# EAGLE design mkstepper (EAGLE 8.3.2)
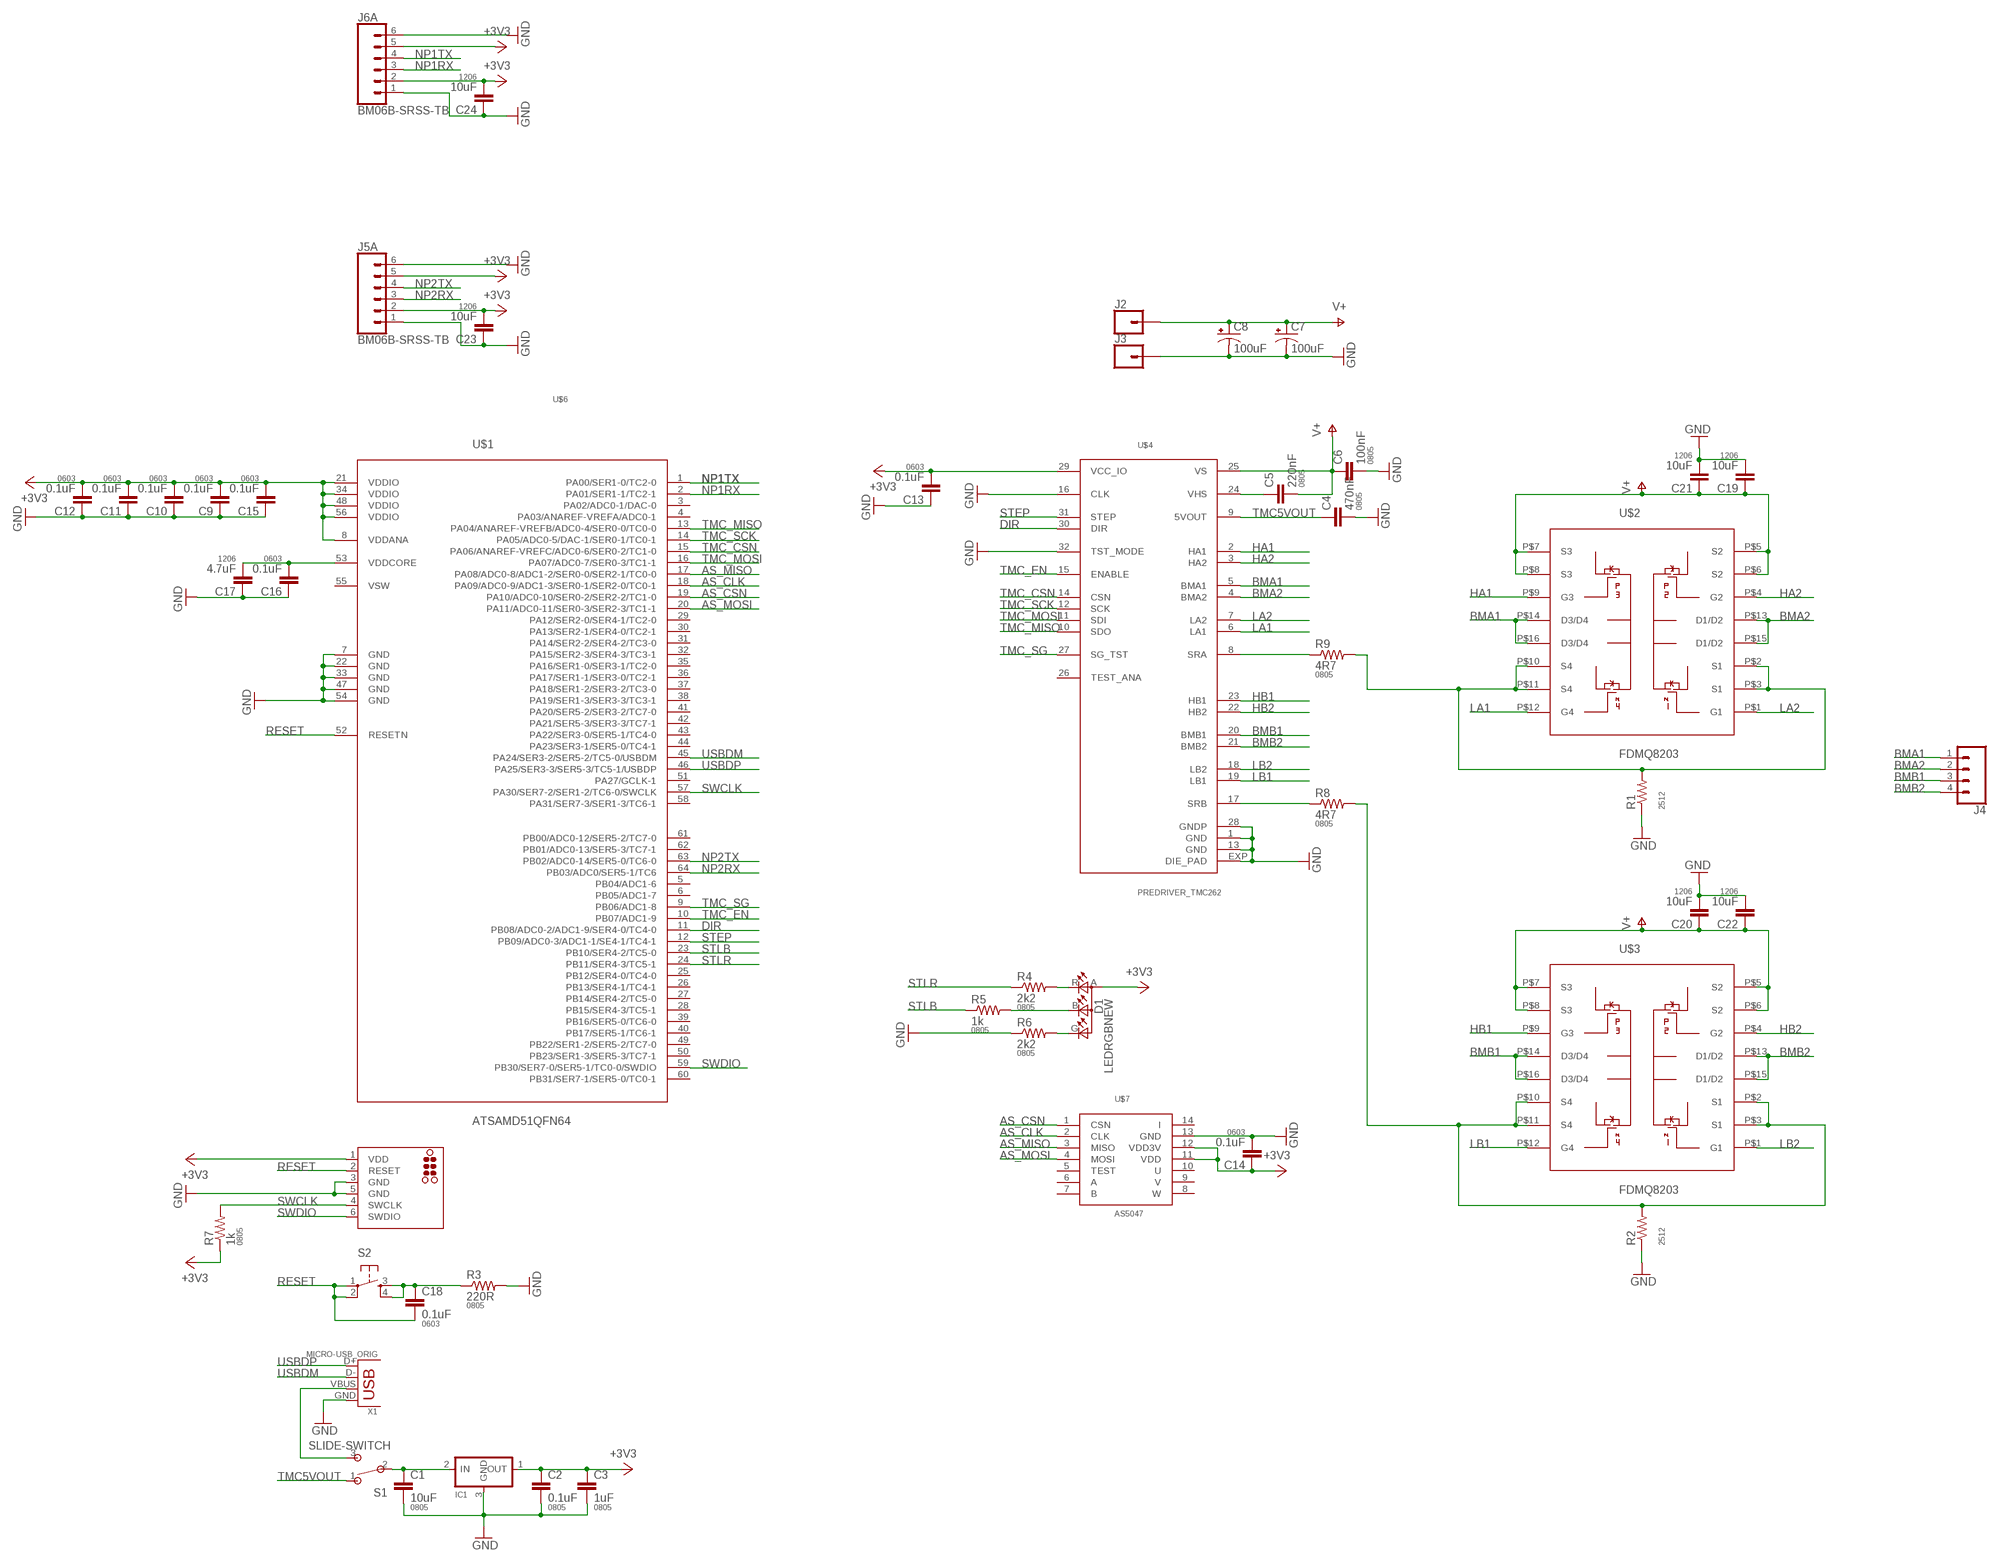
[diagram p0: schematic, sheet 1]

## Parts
C1  10uF  CAP0805  [0805]
C2  0.1uF  CAP0805  [0805]
C3  1uF  CAP0805  [0805]
C4  470nF  CAP0805  [0805]
C5  220nF  CAP0805  [0805]
C6  100nF  CAP0805  [0805]
C7  100uF  CAP-POL-6.6X6.6  [6.6X6.6-CAP]
C8  100uF  CAP-POL-6.6X6.6  [6.6X6.6-CAP]
C9  0.1uF  CAP0603-CAP  [0603-CAP]
C10  0.1uF  CAP0603-CAP  [0603-CAP]
C11  0.1uF  CAP0603-CAP  [0603-CAP]
C12  0.1uF  CAP0603-CAP  [0603-CAP]
C13  0.1uF  CAP0603-CAP  [0603-CAP]
C14  0.1uF  CAP0603-CAP  [0603-CAP]
C15  0.1uF  CAP0603-CAP  [0603-CAP]
C16  0.1uF  CAP0603-CAP  [0603-CAP]
C17  4.7uF  CAP1206  [1206]
C18  0.1uF  CAP0603-CAP  [0603-CAP]
C19  10uF  CAP1206  [1206]
C20  10uF  CAP1206  [1206]
C21  10uF  CAP1206  [1206]
C22  10uF  CAP1206  [1206]
C23  10uF  CAP1206  [1206]
C24  10uF  CAP1206  [1206]
D1  LEDRGBNEW  [P-LCC-4]
IC1  REGULATORSOT23  [SOT23]
J1  TC2030-SWD-MCP  [TC2030-MCP]
J2  CONN_01PTH_2MM  [1X01_2MM]
J3  CONN_01PTH_2MM  [1X01_2MM]
J4  CONN_04LONGPADS  [1X04_LONGPADS]
J5  BM06B-SRSS-TB  JST_6_PIN_HORIZONTAL  [JST-6-SMD-HORI-1.0MM]
J6  BM06B-SRSS-TB  JST_6_PIN_HORIZONTAL  [JST-6-SMD-HORI-1.0MM]
R1  RESISTOR2512  [R2512]
R2  RESISTOR2512  [R2512]
R3  220R  RESISTOR0805-RES  [0805]
R4  2k2  RESISTOR0805-RES  [0805]
R5  1k  RESISTOR0805-RES  [0805]
R6  2k2  RESISTOR0805-RES  [0805]
R7  1k  RESISTOR0805-RES  [0805]
R8  4R7  RESISTOR0805-RES  [0805]
R9  4R7  RESISTOR0805-RES  [0805]
S1  SLIDE-SWITCH  [AYZ0102AGRLC]
S2  6MM_SWITCH6MM_SWITCH  [6MM_SWITCH]
U$1  ATSAMD51QFN64  [QFN-64-9X9MM]
U$2  FDMQ8203  [MLP4.5X5_4PAD]
U$3  FDMQ8203  [MLP4.5X5_4PAD]
U$4  PREDRIVER_TMC262  [QFN32]
U$6  NEMA17  [NEMA17]
U$7  AS5047  [TSSOP14]
X1  MICRO-USB_ORIG  [DX4R005HJ5]

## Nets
+3V3: C2.1 C3.1 C9.2 C10.2 C11.2 C12.2 C13.2 C14.1 C15.2 C23.2 C24.2 D1.A(A2) IC1.1(OUT) J1.1(VDD) J5.2 J5.5 J6.2 J6.5 R7.1 U$1.8(VDDANA) U$1.21(VDDIO) U$1.34(VDDIO) U$1.48(VDDIO) U$1.56(VDDIO) U$4.29(VCC_IO) U$7.11(VDD) U$7.12(VDD3V)
AS_CLK: U$1.18(PA09/ADC0-9/ADC1-3/SER0-1/SER2-0/TC0-1) U$7.2(CLK)
AS_CSN: U$1.19(PA10/ADC0-10/SER0-2/SER2-2/TC1-0) U$7.1(CSN)
AS_MISO: U$1.17(PA08/ADC0-8/ADC1-2/SER0-0/SER2-1/TC0-0) U$7.3(MISO)
AS_MOSI: U$1.20(PA11/ADC0-11/SER0-3/SER2-3/TC1-1) U$7.4(MOSI)
BMA1: J4.1 U$2.P$14(D3/D4) U$2.P$16(D3/D4) U$4.5(BMA1)
BMA2: J4.2 U$2.P$13(D1/D2) U$2.P$15(D1/D2) U$4.4(BMA2)
BMB1: J4.3 U$3.P$14(D3/D4) U$3.P$16(D3/D4) U$4.20(BMB1)
BMB2: J4.4 U$3.P$13(D1/D2) U$3.P$15(D1/D2) U$4.21(BMB2)
DIR: U$1.11(PB08/ADC0-2/ADC1-9/SER4-0/TC4-0) U$4.30(DIR)
GND: C1.2 C2.2 C3.2 C4.2 C6.2 C7.- C8.- C9.1 C10.1 C11.1 C12.1 C13.1 C14.2 C15.1 C16.1 C17.1 C19.2 C20.2 C21.2 C22.2 C23.1 C24.1 IC1.3(GND) J1.3(GND) J1.5(GND) J3.1 J5.1 J5.6 J6.1 J6.6 R1.1 R2.1 R3.2 R6.1 U$1.7(GND) U$1.22(GND) U$1.33(GND) U$1.47(GND) U$1.54(GND) U$4.1(GND) U$4.13(GND) U$4.16(CLK) U$4.28(GNDP) U$4.32(TST_MODE) U$4.EXP(DIE_PAD) U$7.13(GND) X1.GND
HA1: U$2.P$9(G3) U$4.2(HA1)
HA2: U$2.P$4(G2) U$4.3(HA2)
HB1: U$3.P$9(G3) U$4.23(HB1)
HB2: U$3.P$4(G2) U$4.22(HB2)
LA1: U$2.P$12(G4) U$4.6(LA1)
LA2: U$2.P$1(G1) U$4.7(LA2)
LB1: U$3.P$12(G4) U$4.19(LB1)
LB2: U$3.P$1(G1) U$4.18(LB2)
N$1: D1.G(CGREEN) R6.2
N$2: C5.1 U$4.24(VHS)
N$3: C1.1 IC1.2(IN) S1.2
N$4: S1.3 X1.VBUS
N$5: D1.B(CBLUE) R5.2
N$6: D1.R(CRED) R4.2
N$7: C16.2 C17.2 U$1.53(VDDCORE)
N$8: C18.1 R3.1 S2.3(S) S2.4(S1)
N$9: R2.2 R8.2 U$3.P$2(S1) U$3.P$3(S1) U$3.P$10(S4) U$3.P$11(S4)
N$10: R9.1 U$4.8(SRA)
N$11: R8.1 U$4.17(SRB)
N$12: R1.2 R9.2 U$2.P$2(S1) U$2.P$3(S1) U$2.P$10(S4) U$2.P$11(S4)
NP1RX: J6.3 U$1.2(PA01/SER1-1/TC2-1)
NP1TX: J6.4 U$1.1(PA00/SER1-0/TC2-0)
NP2RX: J5.3 U$1.64(PB03/ADC0/SER5-1/TC6)
NP2TX: J5.4 U$1.63(PB02/ADC0-14/SER5-0/TC6-0)
RESET: C18.2 J1.2(RESET) S2.1(P) S2.2(P1) U$1.52(RESETN)
STEP: U$1.12(PB09/ADC0-3/ADC1-1/SE4-1/TC4-1) U$4.31(STEP)
STLB: R5.1 U$1.23(PB10/SER4-2/TC5-0)
STLR: R4.1 U$1.24(PB11/SER4-3/TC5-1)
SWCLK: J1.4(SWCLK) R7.2 U$1.57(PA30/SER7-2/SER1-2/TC6-0/SWCLK)
SWDIO: J1.6(SWDIO) U$1.59(PB30/SER7-0/SER5-1/TC0-0/SWDIO)
TMC5VOUT: C4.1 S1.1 U$4.9(5VOUT)
TMC_CSN: U$1.15(PA06/ANAREF-VREFC/ADC0-6/SER0-2/TC1-0) U$4.14(CSN)
TMC_EN: U$1.10(PB07/ADC1-9) U$4.15(ENABLE)
TMC_MISO: U$1.13(PA04/ANAREF-VREFB/ADC0-4/SER0-0/TC0-0) U$4.10(SDO)
TMC_MOSI: U$1.16(PA07/ADC0-7/SER0-3/TC1-1) U$4.11(SDI)
TMC_SCK: U$1.14(PA05/ADC0-5/DAC-1/SER0-1/TC0-1) U$4.12(SCK)
TMC_SG: U$1.9(PB06/ADC1-8) U$4.27(SG_TST)
USBDM: U$1.45(PA24/SER3-2/SER5-2/TC5-0/USBDM) X1.D-
USBDP: U$1.46(PA25/SER3-3/SER5-3/TC5-1/USBDP) X1.D+
V+: C5.2 C6.1 C7.+ C8.+ C19.1 C20.1 C21.1 C22.1 J2.1 U$2.P$5(S2) U$2.P$6(S2) U$2.P$7(S3) U$2.P$8(S3) U$3.P$5(S2) U$3.P$6(S2) U$3.P$7(S3) U$3.P$8(S3) U$4.25(VS)
Unconnected: J5.M1 J5.M2 J6.M1 J6.M2 U$1.3(PA02/ADC0-1/DAC-0) U$1.4(PA03/ANAREF-VREFA/ADC0-1) U$1.5(PB04/ADC1-6) U$1.6(PB05/ADC1-7) U$1.25(PB12/SER4-0/TC4-0) U$1.26(PB13/SER4-1/TC4-1) U$1.27(PB14/SER4-2/TC5-0) U$1.28(PB15/SER4-3/TC5-1) U$1.29(PA12/SER2-0/SER4-1/TC2-0) U$1.30(PA13/SER2-1/SER4-0/TC2-1) U$1.31(PA14/SER2-2/SER4-2/TC3-0) U$1.32(PA15/SER2-3/SER4-3/TC3-1) U$1.35(PA16/SER1-0/SER3-1/TC2-0) U$1.36(PA17/SER1-1/SER3-0/TC2-1) U$1.37(PA18/SER1-2/SER3-2/TC3-0) U$1.38(PA19/SER1-3/SER3-3/TC3-1) U$1.39(PB16/SER5-0/TC6-0) U$1.40(PB17/SER5-1/TC6-1) U$1.41(PA20/SER5-2/SER3-2/TC7-0) U$1.42(PA21/SER5-3/SER3-3/TC7-1) U$1.43(PA22/SER3-0/SER5-1/TC4-0) U$1.44(PA23/SER3-1/SER5-0/TC4-1) U$1.49(PB22/SER1-2/SER5-2/TC7-0) U$1.50(PB23/SER1-3/SER5-3/TC7-1) U$1.51(PA27/GCLK-1) U$1.55(VSW) U$1.58(PA31/SER7-3/SER1-3/TC6-1) U$1.60(PB31/SER7-1/SER5-0/TC0-1) U$1.61(PB00/ADC0-12/SER5-2/TC7-0) U$1.62(PB01/ADC0-13/SER5-3/TC7-1) U$4.26(TEST_ANA) U$7.5(TEST) U$7.6(A) U$7.7(B) U$7.8(W) U$7.9(V) U$7.10(U) U$7.14(I)

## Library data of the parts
C1-C6 = borkedlabs-passives:CAP: Capacitor; PACKAGE: 0805
C7 C8 = borkedlabs-passives:CAP-POL
C9-C16 C18 = borkedlabs-passives:CAP: Capacitor; PACKAGE: 0603
C17 C19-C24 = borkedlabs-passives:CAP: Capacitor; PACKAGE: 1206
D1 = fab:LEDRGBNEW
IC1 = fab:REGULATOR
J1 = atsam:TC2030-SWD: TAG-CONNECT ICSP Connector Manufacturer: Tag-Connect Cable for easy In-Circuit Serial Programming. Designed for Microchip ICD2, suitable for many others. Two variants - one "with legs" (for hands-free fit on PCB) and another "without legs" for quick programming. PADDescription 1MCLR/Vpp 2Vdd 3GND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
J2 J3 = SparkFun-Connectors:CONN_01: Single connection point. Often used as Generic Header-pin footprint for 0.1 inch spaced/style header connections
J4 = SparkFun-Connectors:CONN_04: Multi connection point. Often used as Generic Header-pin footprint for 0.1 inch spaced/style header connections On any of the 0.1 inch spaced packages, you can populate with these: Break Away Headers - Straight (PRT-00116) Break Away Male Headers - Right Angle (PRT-00553) Female Headers (PRT-00115)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; PROD_ID: CONN-09696
J5 J6 = SparkFun-Connectors:JST_6_PIN_HORIZONTAL: JST 6 pin horizontal connector JST-SH type. Here is the connector we sell at SparkFun: name (XXX-00000) Datasheet It was used on these SparkFun products: name (XXX-00000) name (XXX-00000); PROD_ID: XXX-00000
R1 R2 = borkedlabs-passives:RESISTOR: Resistor; PACKAGE: 2512
R3-R9 = borkedlabs-passives:RESISTOR: Resistor; PACKAGE: 0805
S1 = fab:SLIDE-SWITCH: SMD slide-switch AYZ0102AGRLC as found in the fablab inventory. Includes the mounting holes. Made by Zaerc.
S2 = fab:6MM_SWITCH: OMRON SWITCH
U$1 = atsam:ATSAMD51
U$2 U$3 = power:FDMQ8203
U$4 = power:PREDRIVER_TMC262
U$6 = motors:NEMA17
U$7 = sensor:AS5047
X1 = fab:MICRO-USB: SMD micro USB connector as found in the fablab inventory. Three footprint variants included: original, as described by manufacturer's datasheet for milling with the 1/100" bit for milling with the 1/64" bit Made by Zaerc.

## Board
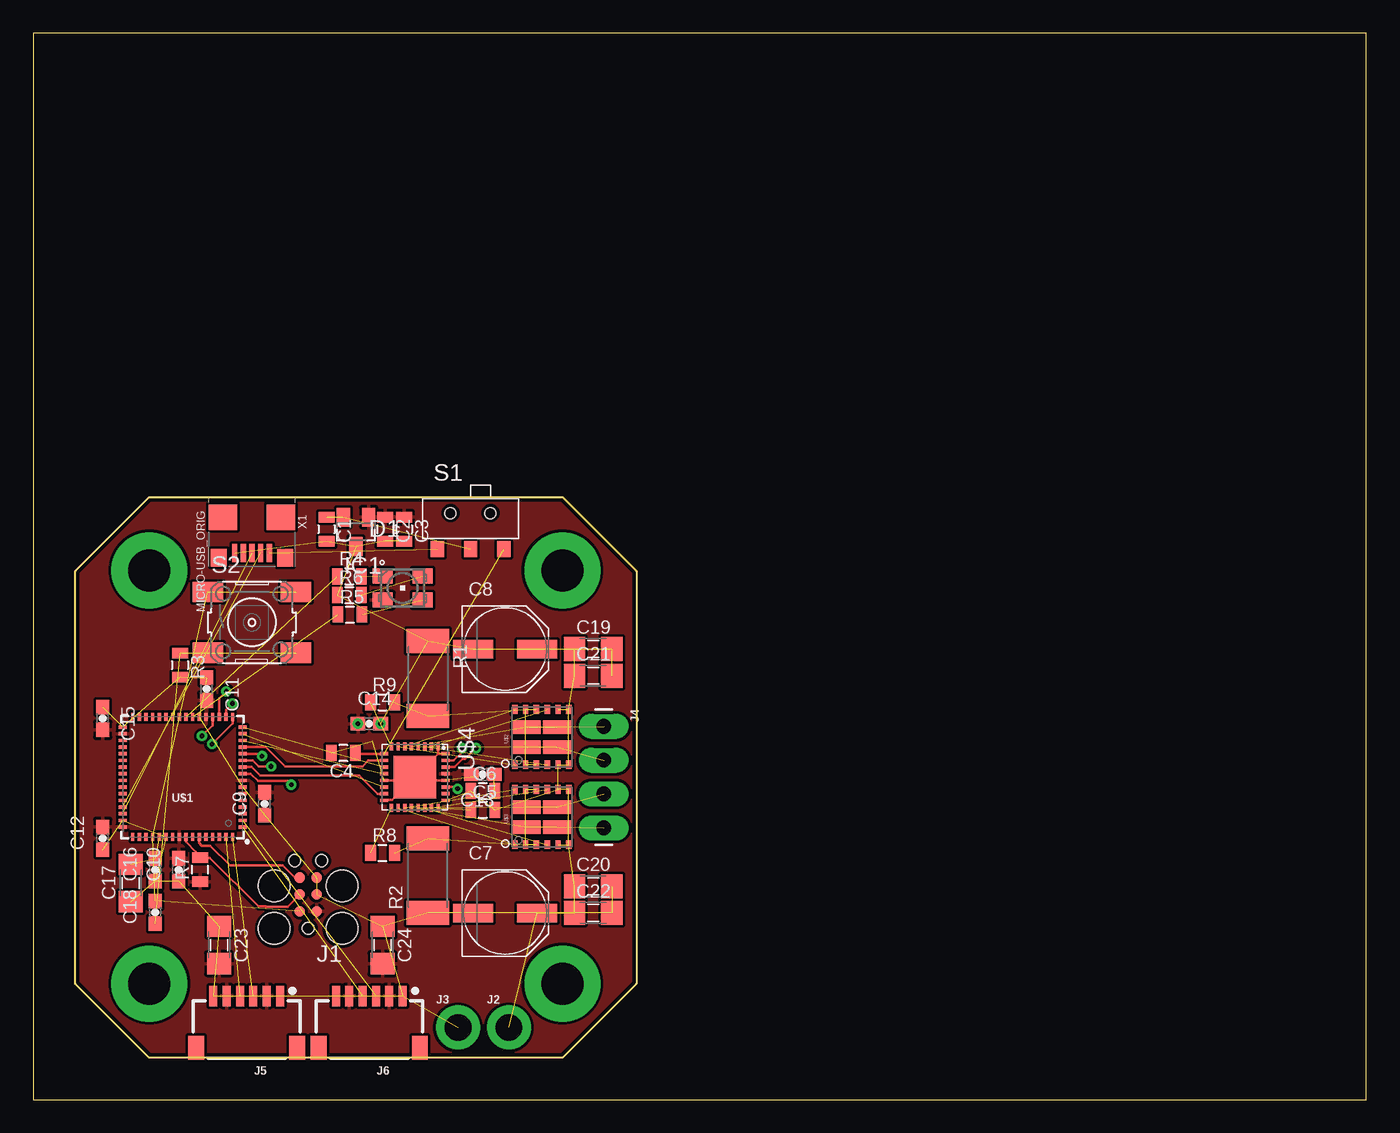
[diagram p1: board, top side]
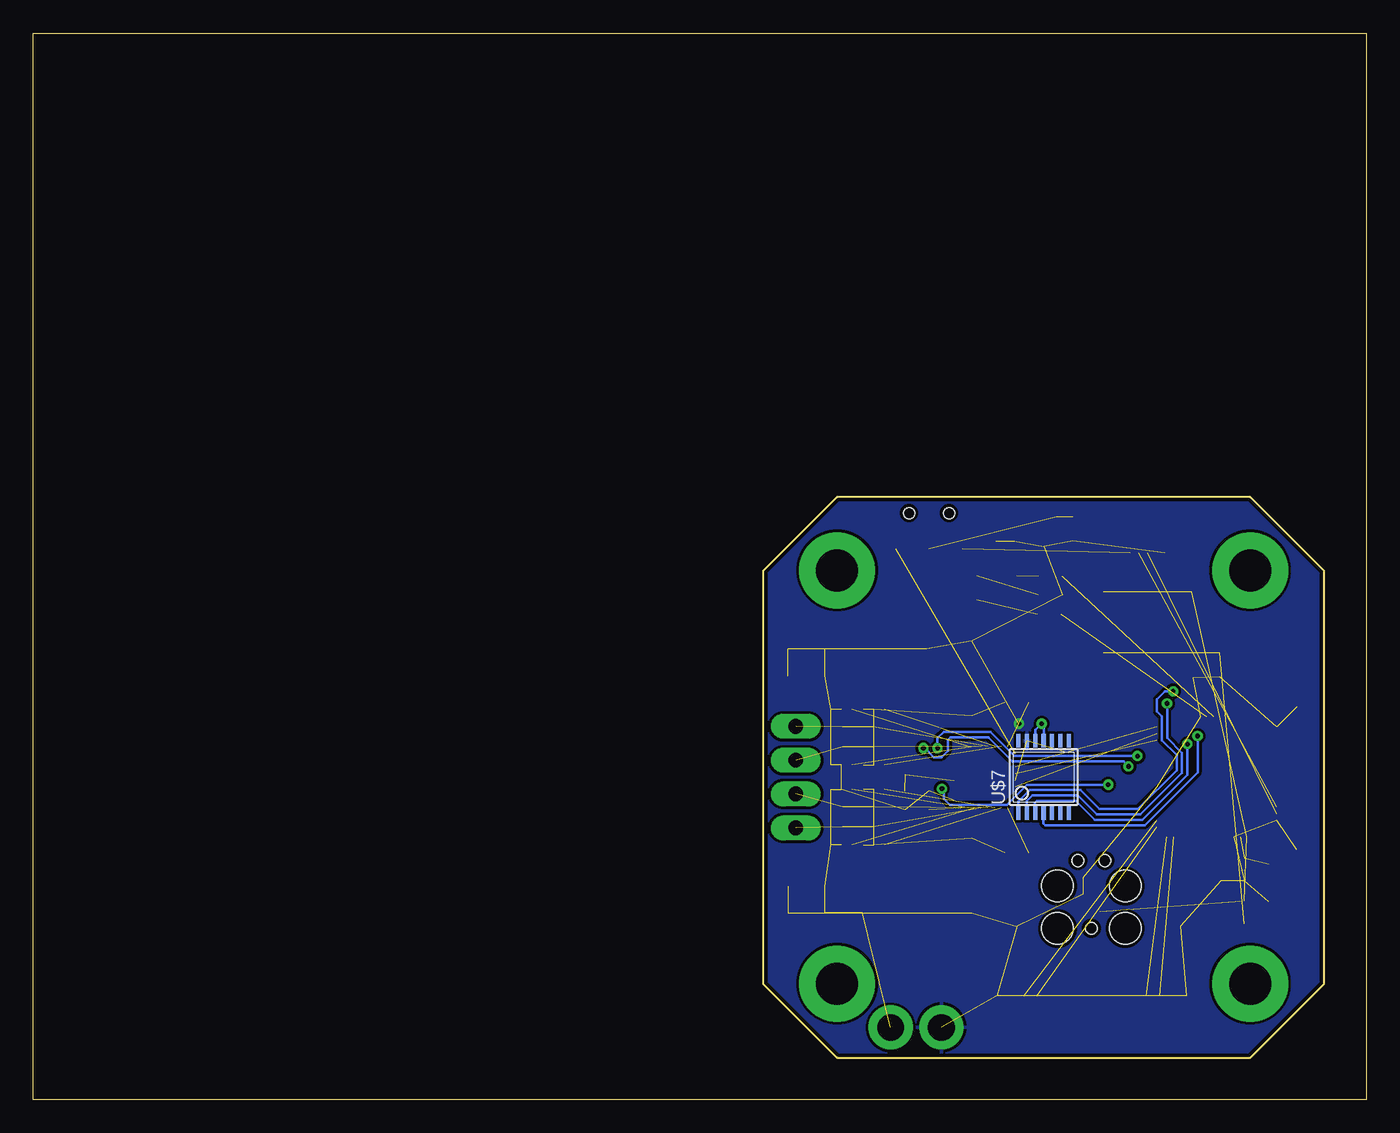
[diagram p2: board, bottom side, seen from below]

Size 100 x 80 mm. Coordinates in mm from the lower left corner, seen from the top.
Outline: 3.15,8.65 3.15,8.7
Outline: 3.15,8.7 3.15,39.65 8.7,45.2 39.7,45.2 45.25,39.65 45.25,8.7 39.7,3.15 8.7,3.15 3.15,8.7
Outline: 0,0 100,0 100,80 0,80 0,0
Copper layers (1*16): Top 0.035mm / dielectric 1.5mm / Bottom 0.035mm
Design rules "default *": minimum track width 6mil, minimum drill 0.35mm, track to track 8mil, track to pad 8mil, pad to pad 8mil, via to via 8mil, smd to smd 8mil, copper to edge 10mil, drill to drill 10mil, minimum pad ring 10mil, minimum via ring 8mil, stop-mask expansion 4mil, vias tented up to drill 20mil, thermal gap 9mil

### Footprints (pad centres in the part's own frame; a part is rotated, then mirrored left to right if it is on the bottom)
0805 = smd 0.8 x 1.2: 1 -0.9,0; 2 0.9,0
6.6X6.6-CAP = smd 3 x 1.4: + 2.4,0; - -2.4,0
0603-CAP = smd 1.1 x 1: 1 -0.85,0; 2 0.85,0
1206 = smd 1.6 x 1.8: 1 -1.4,0; 2 1.4,0
P-LCC-4 = smd 1.1 x 1.5: A 0.902,-1.5; B 0.902,1.5; G -0.902,1.5; R -0.902,-1.5
SOT23 = smd 1 x 1.4: 1 -0.95,-1.1; 2 0.95,-1.1; 3 0,1.1
TC2030-MCP = smd 0.787 x 0.787: 1 1.27,-0.635; 2 1.27,0.635; 3 2.54,-0.635; 4 2.54,0.635; 5 3.81,-0.635; 6 3.81,0.635 | hole 0.889: 0,0; 5.08,-1.016; 5.08,1.016 | hole 2.375: 0,2.54; 0,-2.54; 3.175,-2.54; 3.175,2.54
1X01_2MM = drill 2 pad 3.302: 1 0,0
1X04_LONGPADS = drill 1.118 pad 1.88 long: 1 0,0; 2 2.54,0; 3 5.08,0; 4 7.62,0
JST-6-SMD-HORI-1.0MM = smd 0.6 x 1.55: 1 -2.5,-4.775; 2 -1.5,-4.775; 3 -0.5,-4.775; 4 0.5,-4.775; 5 1.5,-4.775; 6 2.5,-4.775 | smd 1.2 x 1.8: M1 -3.8,-0.9; M2 3.8,-0.9
R2512 = smd 1.8 x 3.2: 1 -2.8,0; 2 2.8,0
AYZ0102AGRLC = smd 1 x 1.2: 1 2.5,-2.3; 2 0,-2.3; 3 -2.5,-2.3 | hole 0.85: -1.5,0.4; 1.5,0.4
6MM_SWITCH = smd 2.286 x 1.524: 1 -3.302,2.286; 2 3.302,2.286; 3 -3.302,-2.286; 4 3.302,-2.286
QFN-64-9X9MM = smd 0.6 x 0.25: 1 -4.5,3.75; 2 -4.5,3.25; 3 -4.5,2.75; 4 -4.5,2.25; 5 -4.5,1.75; 6 -4.5,1.25; 7 -4.5,0.75; 8 -4.5,0.25; 9 -4.5,-0.25; 10 -4.5,-0.75; 11 -4.5,-1.25; 12 -4.5,-1.75; 13 -4.5,-2.25; 14 -4.5,-2.75; 15 -4.5,-3.25; 16 -4.5,-3.75; 33 4.5,-3.75; 34 4.5,-3.25; 35 4.5,-2.75; 36 4.5,-2.25; 37 4.5,-1.75; 38 4.5,-1.25; 39 4.5,-0.75; 40 4.5,-0.25; 41 4.5,0.25; 42 4.5,0.75; 43 4.5,1.25; 44 4.5,1.75; 45 4.5,2.25; 46 4.5,2.75; 47 4.5,3.25; 48 4.5,3.75 | smd 0.25 x 0.6: 17 -3.75,-4.5; 18 -3.25,-4.5; 19 -2.75,-4.5; 20 -2.25,-4.5; 21 -1.75,-4.5; 22 -1.25,-4.5; 23 -0.75,-4.5; 24 -0.25,-4.5; 25 0.25,-4.5; 26 0.75,-4.5; 27 1.25,-4.5; 28 1.75,-4.5; 29 2.25,-4.5; 30 2.75,-4.5; 31 3.25,-4.5; 32 3.75,-4.5; 49 3.75,4.5; 50 3.25,4.5; 51 2.75,4.5; 52 2.25,4.5; 53 1.75,4.5; 54 1.25,4.5; 55 0.75,4.5; 56 0.25,4.5; 57 -0.25,4.5; 58 -0.75,4.5; 59 -1.25,4.5; 60 -1.75,4.5; 61 -2.25,4.5; 62 -2.75,4.5; 63 -3.25,4.5; 64 -3.75,4.5
MLP4.5X5_4PAD = smd 0.4 x 0.65: P$1 -2.02,-2.075; P$2 -1.22,-2.075; P$3 -0.42,-2.075; P$4 0.42,-2.075; P$5 1.22,-2.075; P$6 2.02,-2.075; P$7 2.02,2.075; P$8 1.22,2.075; P$9 0.42,2.075; P$10 -0.42,2.075; P$11 -1.22,2.075; P$12 -2.02,2.075 | smd 2.1 x 1: P$13 1.142,-0.75; P$14 1.142,0.75; P$15 -1.142,-0.75; P$16 -1.142,0.75
QFN32 = smd 0.6 x 0.25: 1 -2.3,1.75; 2 -2.3,1.25; 3 -2.3,0.75; 4 -2.3,0.25; 5 -2.3,-0.25; 6 -2.3,-0.75; 7 -2.3,-1.25; 8 -2.3,-1.75; 17 2.3,-1.75; 18 2.3,-1.25; 19 2.3,-0.75; 20 2.3,-0.25; 21 2.3,0.25; 22 2.3,0.75; 23 2.3,1.25; 24 2.3,1.75 | smd 0.25 x 0.6: 9 -1.75,-2.3; 10 -1.25,-2.3; 11 -0.75,-2.3; 12 -0.25,-2.3; 13 0.25,-2.3; 14 0.75,-2.3; 15 1.25,-2.3; 16 1.75,-2.3; 25 1.75,2.3; 26 1.25,2.3; 27 0.75,2.3; 28 0.25,2.3; 29 -0.25,2.3; 30 -0.75,2.3; 31 -1.25,2.3; 32 -1.75,2.3 | smd 3.2 x 3.2: EXP 0,0
NEMA17 = drill 3.15 pad 5.7: P$1 -15.5,15.5; P$2 15.5,15.5; P$3 -15.5,-15.5; P$4 15.5,-15.5
TSSOP14 = smd 0.305 x 0.991: 1 -1.905,-2.718; 2 -1.27,-2.718; 3 -0.635,-2.718; 4 0,-2.718; 5 0.635,-2.718; 6 1.27,-2.718; 7 1.905,-2.718; 8 1.905,2.718; 9 1.27,2.718; 10 0.635,2.718; 11 0,2.718; 12 -0.635,2.718; 13 -1.27,2.718; 14 -1.905,2.718
DX4R005HJ5 = smd 0.4 x 1.35: D+ 0,1.6; D- -0.65,1.6; GND 1.3,1.6; ID 0.65,1.6; VBUS -1.3,1.6 | smd 1.2 x 1.3: GND@1 -2.5,1.95; GND@2 2.5,1.95 | smd 2.15 x 1.9: GND@3 -2.175,-1.1; GND@4 2.175,-1.1

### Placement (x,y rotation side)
C1  22,42.8 270 top
C2  26.4,42.8 270 top
C3  27.8,42.8 270 top
C4  23.26,26 180 top
C5  33.71,21.74 0 top
C6  33.71,23.14 0 top
C7  35.4,14 0 top
C8  35.4,33.8 0 top
C9  17.35,22.19 90 top
C10  10.9,17.25 90 top
C11  13,30.8 270 top
C12  5.2,19.6 90 top
C13  33.71,24.39 180 top
C14  25.2,28.2 0 top
C15  5.2,28.6 270 top
C16  9.15,17.25 90 top
C17  7.3,16.25 90 top
C18  9.15,14.05 90 top
C19  42,33.8 0 top
C20  42,16 0 top
C21  42,31.8 0 top
C22  42,14 0 top
C23  13.93,11.6 270 top
C24  26.2,11.6 270 top
D1  27.71,38.38 270 top
IC1  24.2,42.6 180 top
J1  20.62,12.84 90 top
J2  35.68,5.41 0 top
J3  31.86,5.41 0 top
J4  42.8,28 270 top
J5  16,3 180 top
J6  25.2,3 180 top
R1  29.6,31.6 270 top
R2  29.6,16.8 90 top
R3  11,32.6 270 top
R4  23.71,39.26 0 top
R5  23.76,36.38 0 top
R6  23.71,37.85 0 top
R7  12.5,17.25 90 top
R8  26.2,18.5 0 top
R9  26.2,29.8 0 top
S1  32.8,43.6 0 top
S2  16.4,35.8 0 top
U$1  11.2,24.2 180 top
U$2  38.15,27.2 0 top
U$3  38.15,21.2 0 top
U$4  28.62,24.19 270 top
U$6  24.2,24.2 0 top
U$7  24.2,24.2 0 bottom
X1  16.4,42.6 180 top

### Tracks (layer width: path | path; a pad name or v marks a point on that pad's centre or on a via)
+3V3  (via drill 0.35)
  Bottom 0.203: U$7.11 24.2,28.05 C14.1 24.84,27.71 U$7.12
  other vias: 24.35,28.2
  pour Top: 3.15,39.65 8.7,45.2 39.7,45.2 45.25,39.65 45.25,8.7 39.7,3.15 8.7,3.15 3.15,8.7
AS_CLK  (via drill 0.35)
  Top 0.203: U$1.18 14.45,29.23 v14.94,29.72
  Bottom 0.203: U$7.2 25.45,21.5 25.45,22.4 25.04,22.81 21.62,22.81 20.2,21.39 16.95,21.39 13.82,24.52 13.82,26.01 14.94,27.13 v14.94,29.72
AS_CSN  (via drill 0.35)
  Top 0.203: U$1.19 13.95,30.1 v14.48,30.63
  Bottom 0.203: U$7.1 26.11,22.36 25.25,23.22 21.46,23.22 20.03,21.79 17.12,21.79 14.22,24.69 14.22,25.84 15.34,26.96 15.34,28.75 15.7,29.11 15.7,30.02 15.09,30.63 v14.48,30.63
AS_MISO  (via drill 0.35)
  Top 0.203: U$1.17 14.95,28.21 v13.41,26.67
  Bottom 0.203: v13.41,26.67 13.41,24.35 16.78,20.98 20.37,20.98 21.79,22.4 24.69,22.4 24.84,22.25 U$7.3
AS_MOSI  (via drill 0.35)
  Top 0.203: U$1.20 13.45,28.08 v12.65,27.28
  Bottom 0.203: v12.65,27.28 12.65,24.54 16.61,20.57 24.08,20.57 24.23,20.73 24.23,21.45 U$7.4
BMA1  (3 unrouted)
BMA2  (3 unrouted)
BMB1  (3 unrouted)
BMB2  (3 unrouted)
DIR  (via drill 0.35)
  Top 0.203: U$4.30 31.61,24.94 32.22,25.54 32.4,25.54 v33.22,26.36 | v17.83,24.99 16.92,24.99 16.46,25.45 U$1.11
  Bottom 0.203: v33.22,26.36 33.12,26.36 32.44,25.68 31.87,25.68 31.39,26.16 31.39,26.98 31.19,27.18 28.36,27.18 26.55,25.36 18.2,25.36 v17.83,24.99
GND  (via drill 0.35)  (39 unrouted)
  Top 0.203: U$4.13 28.37,23.94 U$4.EXP | U$4.16 26.56,22.44 26.62,22.49 26.93,22.49 U$4.EXP | U$4.28 28.87,23.94 U$4.EXP | 30.37,25.94 U$4.32 | 30.37,25.94 U$4.EXP | U$4.1 30.37,25.94
  other vias: 26.05,28.2
  pour Bottom: 3.15,39.65 8.7,45.2 39.7,45.2 45.25,39.65 45.25,8.7 39.7,3.15 8.7,3.15 3.15,8.7
HA1  (1 unrouted)
HA2  (1 unrouted)
HB1  (1 unrouted)
HB2  (1 unrouted)
LA1  (1 unrouted)
LA2  (1 unrouted)
LB1  (1 unrouted)
LB2  (1 unrouted)
N$1  (1 unrouted)
N$2  (1 unrouted)
N$3  (2 unrouted)
N$4  (1 unrouted)
N$5  (1 unrouted)
N$6  (1 unrouted)
N$7  (2 unrouted)
N$8  (3 unrouted)
N$9  (5 unrouted)
N$10  (1 unrouted)
N$11  (1 unrouted)
N$12  (5 unrouted)
NP1RX  (1 unrouted)
NP1TX  (1 unrouted)
NP2RX  (1 unrouted)
NP2TX  (1 unrouted)
RESET  (4 unrouted)
  Top 0.203: 9.3,14.92 C18.2
STEP  (via drill 0.35)
  Top 0.203: U$1.12 16.98,25.95 v17.16,25.77 | v32.16,26.36 32.16,26.06 31.55,25.45 30.93,25.45 U$4.31
  Bottom 0.203: v17.16,25.77 26.38,25.77 28.19,27.58 31.7,27.58 32.16,27.13 v32.16,26.36
STLB  (1 unrouted)
STLR  (1 unrouted)
SWCLK
  Top 0.203: U$1.57 11.45,19.34 12.19,18.59 12.19,18.46 R7.2 13.24,18.15 16.92,14.48 17.43,14.48 17.44,14.47 19.07,14.47 J1.4
SWDIO
  Top 0.203: J1.6 19.62,16.65 18.72,17.56 14.75,17.56 13.26,19.05 12.65,19.05 12.45,19.25 U$1.59
TMC5VOUT  (1 unrouted)
  Top 0.203: U$4.9 24.22,25.94 C4.1
TMC_CSN  (1 unrouted)
TMC_EN
  Top 0.203: U$1.10 16.39,24.95 17.02,24.31 24.46,24.31 25.83,22.94 U$4.15
TMC_MISO
  Top 0.203: U$4.10 25.13,25.44 24.69,24.99 18.9,24.99 17.44,26.45 U$1.13
TMC_MOSI  (1 unrouted)
TMC_SCK  (1 unrouted)
TMC_SG  (via drill 0.35)
  Top 0.203: U$4.27 31.71,23.44 v31.83,23.32 | v19.36,23.62 19.07,23.9 16.86,23.9 16.31,24.45 U$1.9
  Bottom 0.203: v19.36,23.62 25.45,23.62 26.98,22.1 31.24,22.1 31.7,22.55 31.7,23.18 v31.83,23.32
USBDM  (1 unrouted)
USBDP  (1 unrouted)
V+  (17 unrouted)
